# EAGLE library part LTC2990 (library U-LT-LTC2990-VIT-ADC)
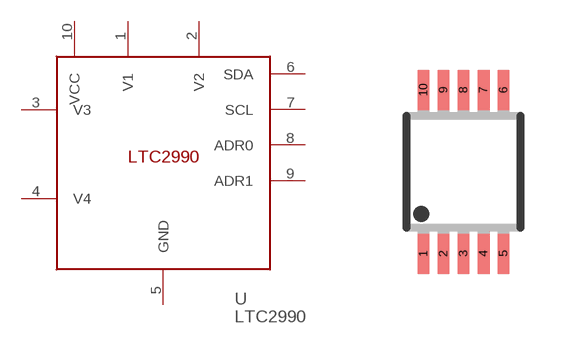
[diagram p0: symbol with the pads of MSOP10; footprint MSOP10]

Designator prefix -

## LTC2990  [MSOP10]
1  V1
2  V2
3  V3
4  V4
5  GND
6  SDA
7  SCL
8  ADR0
9  ADR1
10  VCC

## Footprint MSOP10 (pad centres in mm)
10 Lead Platic MSOP Source: http://www.linear.com .. LT1996
smd 0.3 x 1: 1 -1,-2.05; 2 -0.5,-2.05; 3 0,-2.05; 4 0.5,-2.05; 5 1,-2.05; 6 1,2.05; 7 0.5,2.05; 8 0,2.05; 9 -0.5,2.05; 10 -1,2.05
